PROGRAM P_MAIN_LowSpeed
VAR
	AODB		: ARRAY[0..1] OF ST_IEC870_5_101AODBEntry;(* Application object database including 2 data points *)
	hTable		: T_HAODBTable;(* Application object database handle *)
	fbClient	: FB_IEC870_5_101Master;(* IEC 60870-5-101 master function block instance *)

	nCAA		: DWORD := 7; (* Common ASDU address of remote (slave) station *)

	bSPI		AT%MX0.0 : BOOL;(* Single point information (data point used in monitoring direction slave->master) *)
	bSCS		AT%MX1.5 : BOOL;(* Single command state (data point used in control direction master->slave) *)

	bInit		: BOOL := TRUE;
	nInitErr	: UDINT;
END_VAR

IF bInit THEN
	bInit := FALSE;

	(* Configure protocol parameter *)
	fbClient.protPara.eLinkAddrSize := eIEC870_linkAddr_TwoOctets; (* Link address octet size *)
	fbClient.protPara.linkAddr := 220; (* Link address *)

	(* Configure system parameter *)
	fbClient.sysPara.asduAddr := nCAA; (* Common ASDU address of remote (slave) station *)
	fbClient.sysPara.asduFmt.eCOTSize := eIEC870_COT_TwoOctets;(* Cause of transfer octet size *)
	fbClient.sysPara.asduFmt.eAsduAddrSize := eIEC870_AsduAddr_TwoOctets;(* Common ASDU address octet size *)
	fbClient.sysPara.asduFmt.eObjAddrSize := eIEC870_ObjAddr_ThreeOctets;(* Information object address octet size *)
	fbClient.sysPara.dbgMode := IEC870_DEBUGMODE_DEVSTATE(* OR IEC870_DEBUGMODE_LINKERROR OR IEC870_DEBUGMODE_ASDU OR IEC870_DEBUGMODE_LINKLAYER *); (* Enable debug output of device state change *)


	nInitErr := F_iecCreateTableHnd( ADR( AODB ), SIZEOF( AODB ), hTable );(* Initialize database handle *)


	(* Configure one single point in monitoring direction *)
	nInitErr := F_iecAddTableEntry( M_SP_NA_1, (* Type is single point *)
									nCAA, (* Common ASDU address *)
									100, (* Information object address *)
									IEC870_GRP_INROGEN, (* Interrogation group *)
									0,(* Multiplier (not used) *)
									MAP_AREA_MEMORY,(* Map this single point value TO PLC memory area (buffer) *)
									0, (* Map TO byte offset *)
									0, (* Map TO bit offset *)
									0, (* Not used *)
									hTable );(* Application object database handle *)

	(* Configure one single command in control direction *)
	nInitErr := F_iecAddTableEntry( C_SC_NA_1, (* Type is single command *)
									nCAA, (* Common ASDU address *)
									10,(* Information object address *)
									0, (* Group (not used) *)
									0, (* Multiplier (not used) *)
									MAP_AREA_MEMORY, (* Map this single command value FROM PLC memory area (buffer) *)
									1, (* Map FROM byte offset *)
									5, (* Map FROM bit offset *)
									0, (* Not used *)
									hTable );(* Application object database handle *)

ELSE
	(* Execute IEC master function block *)
	fbClient(	pAOEntries	:= ADR( AODB ),(* Start address of application object database *)
				cbAOEntries := SIZEOF( AODB ),(* Byte size of application object database *)
				pInputs 	:= 0, (* Not used *)
				cbInputs 	:= 0, (* Not used *)
				pOutputs 	:= 0, (* Not used *)
				cbOutputs 	:= 0, (* Not used *)
				pMemory 	:= ADR( %MB0 ),(* Start address of memory area (buffer). Memory buffer where the data point values are mapped to and from *)
				cbMemory 	:= 2,(* Byte size of memory area (buffer) = 2 byte (%MB0..%MB1) *)
				pData 		:= 0, (* Not used *)
				cbData 		:= 0, (* Not used *)
				hTable 		:= hTable,(* Application object database handle *)
				hSerial 	:= P_SerialComm_HighSpeed.hSerial,(* Serial port connection/communication handle *)
				bEnable 	:= TRUE(* Enable communication *) );


	(* Check for device errors, remove them and log errror message to the TwinCAT->Error List CTRL+^, E *)
	REPEAT
		fbClient.system.device.errors.RemoveError( );
		IF fbClient.system.device.errors.bOk THEN
			ADSLOGSTR( ADSLOG_MSGTYPE_ERROR OR ADSLOG_MSGTYPE_LOG, 'IEC60870-5-101 master error: 0x%s',
						DWORD_TO_HEXSTR( fbClient.system.device.errors.getError.nErrId, 8, FALSE) );
		END_IF
	UNTIL NOT fbClient.system.device.errors.bOk
	END_REPEAT

END_IF

END_PROGRAM
